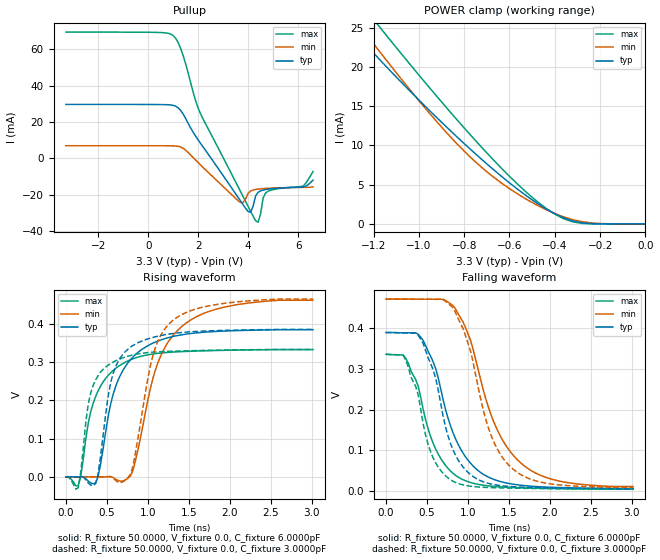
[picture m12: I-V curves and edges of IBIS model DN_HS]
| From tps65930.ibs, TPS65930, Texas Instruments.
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|   Model DN_HS
[Model]  DN_HS
Model_type I/O_open_source
Polarity   Inverting
Enable   Active-High
Vinl =   1.1550V
Vinh =   2.1450V
Vmeas =  0.3000V
Cref =   5.0000pF
Rref =   50.0000
Vref =   0.0V
C_comp   6.1523pF   6.1128pF   6.1708pF
[Temperature Range]   25.0000   0.1250k   -40.0000
[Pullup Reference]   3.3000V   3.0000V   3.6000V
[Pulldown Reference]   0.0V   0.0V   0.0V
[POWER Clamp Reference]   3.3000V   3.0000V   3.6000V
[GND Clamp Reference]   0.0V   0.0V   0.0V
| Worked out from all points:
|   slope of the pullup table from 0 to 0.495 V, typ, clamps not added: 10.8 kohm
|   POWER clamp passes 1 mA (typ) near -0.38 V on its own axis
|   rising waveform, R_fixture 50.0000, V_fixture 0.0, C_fixture 6.0000pF: 20-80 % time 338ps typ, 406ps min, 296ps max; typ from 0 V to 0.385 V
|   rising waveform, R_fixture 50.0000, V_fixture 0.0, C_fixture 3.0000pF: 20-80 % time 220ps typ, 290ps min, 191ps max; typ from 0 V to 0.386 V
|   falling waveform, R_fixture 50.0000, V_fixture 0.0, C_fixture 6.0000pF: 20-80 % time 391ps typ, 479ps min, 327ps max; typ from 0.389 V to 0.006 V
|   falling waveform, R_fixture 50.0000, V_fixture 0.0, C_fixture 3.0000pF: 20-80 % time 317ps typ, 388ps min, 272ps max; typ from 0.389 V to 0.005 V
[Pullup]
|Voltage   I(typ)   I(min)   I(max)
-3.3V     29.62mA    6.891mA    69.41mA
1V        29.11mA    6.815mA    67.45mA
1.3V      26.26mA    6.17mA     60.35mA
2.1V      8.074mA    -3.767mA   24.32mA
3.7V      -23.59mA   -24.36mA   -18.43mA
4V        -29.32mA   -19.25mA   -26.51mA
4.1V      -29.65mA   -18.04mA   -29.21mA
4.4V      -18.73mA   -16.97mA   -35.18mA
4.6V      -17.52mA   -16.71mA   -21.82mA
4.7V      -17.22mA   -16.62mA   -19.13mA
6.2V      -15.78mA   -16.03mA   -15.33mA
6.6V      -12.03mA   -15.68mA   -7.305mA
[POWER_clamp]
|Voltage   I(typ)   I(min)   I(max)
-3.28V    107.5mA    105.3mA    115.4mA
-1.32V    25.64mA    27.45mA    30.4mA
-1.28V    24.31mA    25.93mA    28.93mA
-1.24V    23.01mA    24.43mA    27.48mA
-1.16V    20.52mA    21.45mA    24.6mA
-920mV    13.51mA    12.98mA    16.21mA
-760mV    9.177mA    8.157mA    10.93mA
-600mV    5.228mA    4.491mA    6.062mA
-440mV    1.936mA    1.837mA    2.017mA
-360mV    762.5uA    886.4uA    652.5uA
-280mV    147.6uA    287.8uA    73.11uA
0V        3.69nA     62.74nA    1.774nA
[Ramp]
| variable   typ   min   max
dV/dt_r  0.4475/0.3224n   0.6163/0.5357n   0.3454/0.2254n
dV/dt_f  0.4601/0.3614n   0.6699/0.5835n   0.3471/0.2825n
R_load = 50.0000k
[Rising Waveform]
R_fixture= 50.0000
V_fixture= 0.0
V_fixture_min= 0.0
V_fixture_max= 0.0
C_fixture= 6.0000pF
|time   V(typ)   V(min)   V(max)
0s        -25.64uV   44.95uV    -33.33uV
151.5ps   -8.421uV   -7.938uV   -23.09mV
363.6ps   -15.5mV    11.58uV    210.5mV
575.8ps   215.3mV    -1.813mV   278mV
727.3ps   289.2mV    -7.807mV   300.1mV
818.2ps   313.4mV    16.97mV    308.7mV
1.121ns   355mV      297.5mV    322.9mV
1.394ns   370.7mV    389.4mV    327.3mV
2ns       381.7mV    446.8mV    331.1mV
3.015ns   384.8mV    461.9mV    332.8mV
[Rising Waveform]
R_fixture= 50.0000
V_fixture= 0.0
V_fixture_min= 0.0
V_fixture_max= 0.0
C_fixture= 3.0000pF
|time   V(typ)   V(min)   V(max)
0s        -42.96uV   56.84uV    -50.85uV
151.5ps   -13.94uV   -19.6uV    -28.13mV
272.7ps   -15.98mV   7.706uV    190.5mV
363.6ps   -17.56mV   14.58uV    253.8mV
575.8ps   269.6mV    -3.044mV   300mV
818.2ps   343.5mV    27.93mV    318.8mV
1.061ns   364.5mV    316.3mV    326mV
1.273ns   373.8mV    403mV      328.3mV
1.849ns   382.5mV    451.1mV    331.2mV
3.015ns   385.5mV    464.9mV    333.1mV
[Falling Waveform]
R_fixture= 50.0000
V_fixture= 0.0
V_fixture_min= 0.0
V_fixture_max= 0.0
C_fixture= 6.0000pF
|time   V(typ)   V(min)   V(max)
0s        389.3mV    471.5mV    335.8mV
242.4ps   388.6mV    471.5mV    325.6mV
454.5ps   369.9mV    471.2mV    200.4mV
636.4ps   279mV      471.1mV    90.93mV
757.6ps   178.7mV    464mV      55.13mV
909.1ps   103.6mV    425.9mV    30.58mV
1.303ns   29.12mV    176mV      11.12mV
1.606ns   14.73mV    76mV       7.705mV
2.091ns   8.248mV    25.15mV    5.559mV
3.015ns   5.579mV    10.6mV     4.259mV
[Falling Waveform]
R_fixture= 50.0000
V_fixture= 0.0
V_fixture_min= 0.0
V_fixture_max= 0.0
C_fixture= 3.0000pF
|time   V(typ)   V(min)   V(max)
0s        389.3mV    471.5mV    335.7mV
212.1ps   388.4mV    471.5mV    333mV
393.9ps   382.8mV    471.1mV    235.9mV
454.5ps   362.3mV    471.1mV    164.8mV
606.1ps   277.5mV    471mV      69.07mV
818.2ps   101mV      449.9mV    23.67mV
1.03ns    40.32mV    345.1mV    11.42mV
1.273ns   17.29mV    141.7mV    7.974mV
1.515ns   10.66mV    59.9mV     6.751mV
3.015ns   5.17mV     8.554mV    4.096mV
